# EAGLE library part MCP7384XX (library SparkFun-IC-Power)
Li-Ion charge controller family from Microchip (IC-08344)
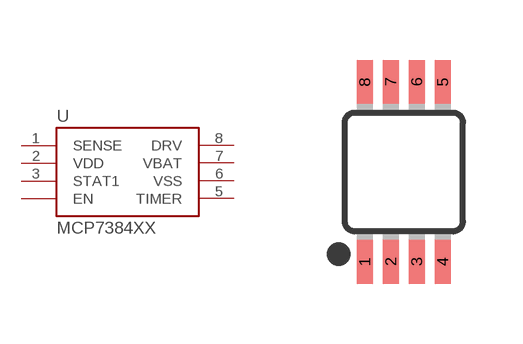
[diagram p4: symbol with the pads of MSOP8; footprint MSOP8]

Designator prefix U

## MCP7384XX  [MSOP8]
1  SENSE
2  VDD
3  STAT1
4  EN
5  TIMER
6  VSS
7  VBAT
8  DRV

## Footprint MSOP8 (pad centres in mm)
8M, 8-Lead, 0.118" Wide, Miniature Small Outline Package MSOP 8M-Package doc1097.pdf
smd 0.4 x 1.1: 1 -0.975,-2.25; 2 -0.325,-2.25; 3 0.325,-2.25; 4 0.975,-2.25; 5 0.975,2.25; 6 0.325,2.25; 7 -0.325,2.25; 8 -0.975,2.25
